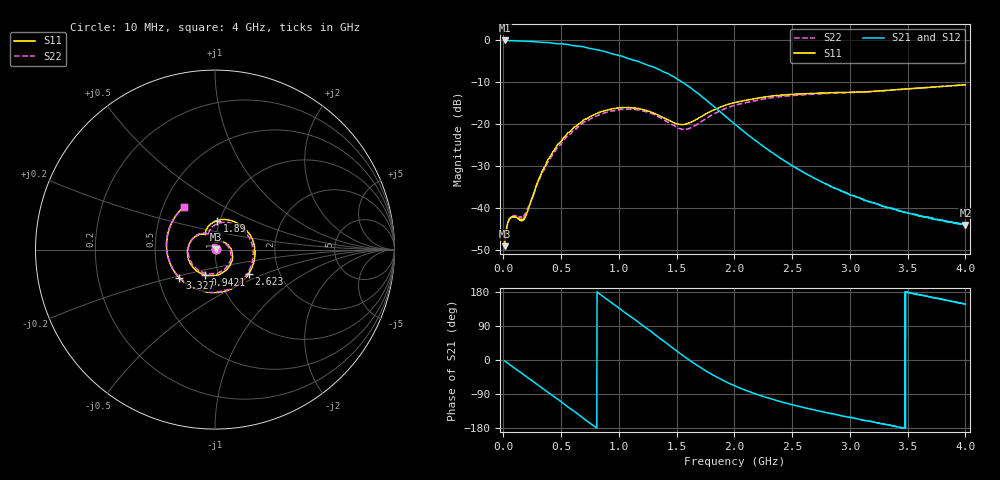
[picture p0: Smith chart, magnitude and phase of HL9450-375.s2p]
! 7/13/2020 7:53:48 AM
! H:\PRODUCTION_DATA\9450\10014\HL9450_10009_933MHZ_.S2P
! CHANNEL.1
! TR.MEASUREMENT
! CORRECTED.DATA
# GHZ S RI R 50.0
! FREQ.GHZ  S11RE  S11IM  S21RE  S21IM  S12RE  S12IM  S22RE  S22IM
!; PortSelection: Port_12
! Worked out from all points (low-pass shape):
!   2000 points, 10 MHz to 4 GHz, reference 50 ohm
!   highest |S21| = -0.03 dB at 10 MHz (marker M1); lowest = -44.1 dB at 4 GHz (marker M2)
!   |S21| within 3 dB of the highest: start of sweep to 919.3 MHz
!   lowest |S11| = -49.1 dB at 10 MHz (marker M3), VSWR 1.01, Z = 50.3 + j0.185 ohm
!   |S11| at or under -10 dB: start of sweep to end of sweep
!   |S22| runs from -49.0 to -10.6 dB; largest |S21 - S12| = 0.0074
!   S11 on the Smith chart (normalised r, x): 10 MHz: 1.01, +0.00; 942.1 MHz: 0.86, -0.25; 1.89 GHz: 0.97, +0.32; 2.623 GHz: 1.40, -0.40; 3.327 GHz: 0.64, -0.22; 4 GHz: 0.64, +0.33
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0.01  0.00298 0.00184  0.9959 -0.0403  0.9974 -0.0404  0.003 0.00189
0.05989995  0.00757 -0.000663  0.965 -0.2301  0.9654 -0.2308  0.00759 -0.000947
0.1876438  -0.00567 -0.00536  0.7322 -0.6478  0.7319 -0.6482  -0.00589 -0.00611
0.3652876  -0.0044 0.0322  0.1597 -0.9327  0.1588 -0.9326  -0.00484 0.0302
0.5129915  0.0538 0.0389  -0.3577 -0.8353  -0.3574 -0.8364  0.0506 0.036
0.6766633  0.0971 -0.0439  -0.7313 -0.4229  -0.7315 -0.4214  0.0889 -0.044
0.8143872  0.0431 -0.1279  -0.7723 0.0139  -0.7697 0.0167  0.0332 -0.1221
0.9421311  -0.0581 -0.1414  -0.599 0.345  -0.5976 0.3473  -0.0651 -0.1277
1.039935  -0.1237 -0.0974  -0.3899 0.5032  -0.3949 0.5006  -0.1265 -0.0812
1.149715  -0.1535 -0.0207  -0.1406 0.5545  -0.1377 0.5492  -0.1487 -0.00368
1.341331  -0.1019 0.0774  0.2231 0.3939  0.2247 0.3909  -0.0851 0.0884
1.576858  -0.0523 0.0852  0.2965 0.0347  0.2966 0.0356  -0.0328 0.0801
1.89023  0.0117 0.1619  0.0832 -0.107  0.0828 -0.1068  0.0183 0.1464
2.005998  0.0742 0.1658  0.0365 -0.0927  0.0361 -0.093  0.0764 0.1502
2.33933  0.2146 0.0388  -0.0111 -0.0431  -0.0112 -0.043  0.207 0.0275
2.622761  0.1877 -0.1351  -0.0154 -0.0204  -0.0153 -0.0205  0.1769 -0.1395
2.670665  0.1696 -0.1594  -0.0153 -0.0179  -0.0152 -0.0179  0.1583 -0.1629
2.984037  -0.00672 -0.2403  -0.0129 -0.00717  -0.0127 -0.00731  -0.0157 -0.2374
3.327349  -0.198 -0.1581  -0.01 -0.00162  -0.00996 -0.00161  -0.2022 -0.1524
3.335333  -0.2016 -0.1543  -0.00995 -0.00147  -0.00999 -0.0015  -0.2055 -0.1485
3.662676  -0.2695 0.0427  -0.00755 0.00149  -0.00765 0.00153  -0.2693 0.0475
4  -0.1735 0.2387  -0.00526 0.0034  -0.0053 0.0034  -0.1714 0.2399
